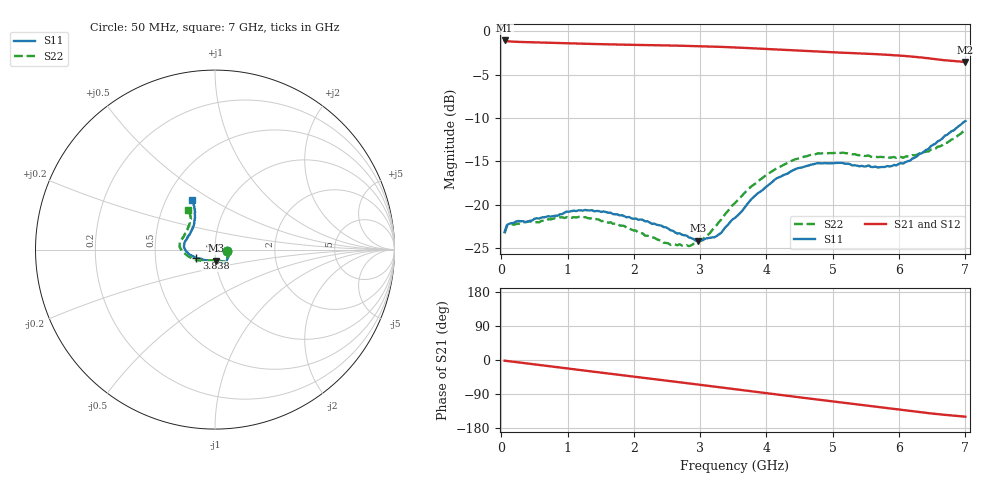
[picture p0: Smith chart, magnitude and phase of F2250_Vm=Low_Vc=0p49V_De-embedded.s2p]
! Integrated Device Technology
! Corporate Headquarters
! 6024 Silver Creek Valley Road
! San Jose, CA 95138  USA
! Phone:  1-408-284-8200
! Toll Free:  1-800-223-1366
! Webpage:  http://www.idt.com/
! Timing and RF Division
! 515 Groton Road, Suite 102
! Westford, MA 01886-6024
! Device:  F2250
! Description: Voltage Variable RF Attenuator
! Frequency:  50.0 -  6000.00 MHz
! Package:  3x3 mm Thin QFN Plastic Package: 16 pin
! Ports:  2 RF, 3 DC
!  Pin  1  = GND
!  Pin  2  = NC
!  Pin  3  = RF1  = Port 1
!  Pin  4  = NC
!  Pin  5  = GND
!  Pin  6  = GND
!  Pin  7  = GND
!  Pin  8  = GND
!  Pin  9  = NC
!  Pin 10  = RF2  = Port 2
!  Pin 11  = NC
!  Pin 12  = GND
!  Pin 13  = GND
!  Pin 14  = VCNTRL
!  Pin 15  = VDD
!  Pin 16  = VMODE
! Vcntrl:  0.490 Volts
! Vmode:  +0.000 Volts
! Vdd:  +3.30  Volts
! Current:  1.128 mA
! Data:  The device was measured on a the F2250 evaluation board which has
!  individual transmission lines to the RF pins.  Data was collected
!  using a calibrated network analyzer.  The evaluation board was
!  de-embedded using a TRL calibration technique.
!  The reference plane is the edge of the package pin.
! Misc:  SN 10
!  Action Tracker AT0258
! Date Measured:  2014-11-26
! Date:  2015-10-15  MJV
! Note:
!  Integrated Device Technology supplies this data as a sample of measured
!  data at the package pin for this product.  Your particular data for this
!  product may vary.
!  Data was taken at 25 degrees C.
!  Integrated Device Technology reserves the right to change this data at anytime.
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# GHz S dB R 50
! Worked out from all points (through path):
!   201 points, 50 MHz to 7 GHz, reference 50 ohm
!   highest |S21| = -1.07 dB at 50 MHz (marker M1); lowest = -3.6 dB at 7 GHz (marker M2)
!   group delay of S21, straight-line fit = 60.1 ps
!   lowest |S11| = -24.1 dB at 2.969 GHz (marker M3), VSWR 1.13, Z = 50.2 - j6.24 ohm
!   |S11| at or under -10 dB: start of sweep to end of sweep
!   |S22| runs from -24.7 to -11.4 dB; largest |S21 - S12| = 0.00041
!   S11 on the Smith chart (normalised r, x): 50 MHz: 1.15, -0.02; 3.838 GHz: 0.81, -0.08; 7 GHz: 0.67, +0.41
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0.05  -23.10 -7.9  -1.07 -1.8  -1.07 -1.8  -23.28 -8.7
0.08475  -22.30 -7.8  -1.15 -2.5  -1.15 -2.5  -22.44 -8.1
0.15425  -22.09 -9.9  -1.19 -4.0  -1.19 -4.0  -22.23 -9.9
0.6755  -21.38 -31.5  -1.32 -15.4  -1.32 -15.4  -21.81 -33.7
0.884  -21.08 -40.2  -1.37 -20.0  -1.36 -20.0  -21.43 -43.6
1.2315  -20.66 -49.9  -1.44 -27.4  -1.44 -27.4  -21.44 -56.1
1.75275  -21.10 -56.7  -1.54 -38.5  -1.53 -38.5  -22.14 -64.6
2.37825  -22.34 -58.4  -1.62 -51.8  -1.62 -51.8  -24.04 -70.1
2.7605  -23.50 -70.7  -1.68 -60.2  -1.68 -60.2  -24.75 -87.4
2.969  -24.13 -85.0  -1.72 -64.8  -1.72 -64.8  -24.27 -103.3
3.247  -23.59 -112.5  -1.79 -71.0  -1.79 -71.0  -22.33 -126.2
3.525  -21.49 -137.9  -1.87 -77.2  -1.87 -77.2  -19.78 -143.3
3.83775  -18.88 -155.8  -1.99 -84.1  -1.99 -84.1  -17.51 -157.3
4.1505  -16.95 -168.1  -2.11 -90.9  -2.12 -90.9  -15.80 -169.4
4.4285  -15.91 -176.3  -2.22 -96.9  -2.22 -97.0  -14.76 -176.8
4.7065  -15.31 176.7  -2.32 -103.0  -2.33 -103.0  -14.22 177.0
5.15825  -15.19 165.8  -2.48 -112.7  -2.48 -112.7  -13.98 167.5
5.85325  -15.58 142.2  -2.73 -127.6  -2.73 -127.6  -14.56 152.0
6.166  -14.90 130.8  -2.90 -134.4  -2.90 -134.5  -14.41 143.1
6.444  -13.56 121.8  -3.11 -140.2  -3.11 -140.3  -13.84 133.6
6.82625  -11.42 115.6  -3.43 -146.9  -3.43 -146.9  -12.40 125.6
7  -10.35 114.8  -3.55 -149.5  -3.55 -149.6  -11.40 124.1
